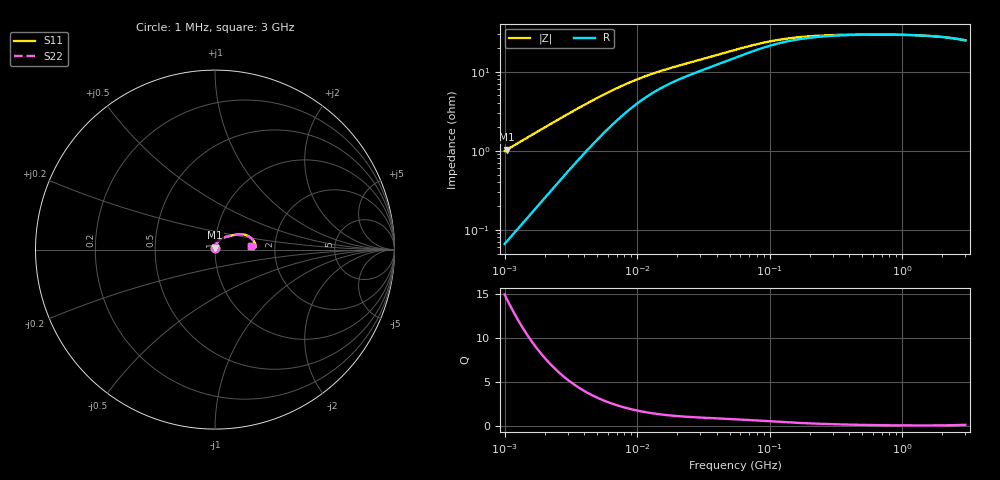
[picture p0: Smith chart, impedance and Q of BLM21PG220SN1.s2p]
! BLM21PG220SN1
# Hz S RI R 50
!Freq.(Hz) S11(Real) S11(Imag) S21(Real) S21(Imag) S12(Real) S12(Imag) S22(Real) S22(Imag)
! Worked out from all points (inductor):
!   401 points, 1 MHz to 3 GHz, reference 50 ohm
!   read as one part in series: L = 157 nH near 1.041 MHz
!   highest Q = 14.4 at 1.041 MHz (marker M1), where L = 157 nH
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1000000  0.00076 0.00988  0.9992 -0.00988  0.9992 -0.00988  0.00076 0.00988
1040844  0.00082 0.0103  0.9992 -0.0103  0.9992 -0.0103  0.00082 0.0103
2271982  0.00368 0.0219  0.9963 -0.0219  0.9963 -0.0219  0.00368 0.0219
3823119  0.0097 0.0348  0.9903 -0.0348  0.9903 -0.0348  0.0097 0.0348
5592179  0.0186 0.0467  0.9814 -0.0467  0.9814 -0.0467  0.0186 0.0467
7703107  0.0302 0.0568  0.9698 -0.0568  0.9698 -0.0568  0.0302 0.0568
9040831  0.0374 0.0613  0.9626 -0.0613  0.9626 -0.0613  0.0374 0.0613
1.061086e7  0.0452 0.0652  0.9548 -0.0652  0.9548 -0.0652  0.0452 0.0652
1.461624e7  0.0619 0.0711  0.9381 -0.0711  0.9381 -0.0711  0.0619 0.0711
2.095589e7  0.0807 0.0756  0.9193 -0.0756  0.9193 -0.0756  0.0807 0.0756
3.526298e7  0.1091 0.0822  0.8909 -0.0822  0.8909 -0.0822  0.1091 0.0822
5.477226e7  0.1385 0.086  0.8615 -0.086  0.8615 -0.086  0.1385 0.086
7.697298e7  0.1639 0.0833  0.8361 -0.0833  0.8361 -0.0833  0.1639 0.0833
1.060286e8  0.1859 0.0747  0.8141 -0.0747  0.8141 -0.0747  0.1859 0.0747
1.460522e8  0.2031 0.0625  0.7969 -0.0625  0.7969 -0.0625  0.2031 0.0625
2.094008e8  0.2156 0.0479  0.7844 -0.0479  0.7844 -0.0479  0.2156 0.0479
3.817355e8  0.2252 0.0284  0.7748 -0.0284  0.7748 -0.0284  0.2252 0.0284
8.005644e8  0.2269 0.0148  0.7731 -0.0148  0.7731 -0.0148  0.2269 0.0148
1.218836e9  0.2241 0.0113  0.7759 -0.0113  0.7759 -0.0113  0.2241 0.0113
1.712864e9  0.2189 0.0112  0.7811 -0.0112  0.7811 -0.0112  0.2189 0.0112
2.266846e9  0.2112 0.014  0.7888 -0.014  0.7888 -0.014  0.2112 0.014
3e9  0.199 0.0221  0.801 -0.0221  0.801 -0.0221  0.199 0.0221
